| v69a.ibs * IBIS 4.1 Model
| 2Gb DDR-3 SDRAM - Die Revision "D"
| This Model is valid for Commercial Temperature Range (0C to 95C)
| Valid for DDR3-800/1066/1333/1600/1866/2133 operation
| Models *_1066 are applicable for speed grade 800/1066 Mbps
| Models *_1333 are applicable for speed grade 1333Mbps
| Models *_1600 are applicable for speed grade 1600Mbps
| Models *_2133 are applicable for speed grade 1866/2133 Mbps
| Part Number   VDD/VDDQ   Architecture   Package
| MT41J512M4HX   1.5V/1.5V   512Meg x 4   78-Ball 9x11.5 FBGA
| MT41J256M8HX   1.5V/1.5V   256Meg x 8   78-Ball 9x11.5 FBGA
| MT41J128M16HA   1.5V/1.5V   128Meg x 16   96-Ball 9x14.0 FBGA
| MT41J512M4V69A   1.5V/1.5V   512Meg x 4   Bare Die
| MT41J256M8V69A   1.5V/1.5V   256Meg x 8   Bare Die
| MT41J128M16V69A   1.5V/1.5V   128Meg x 16   Bare Die
[IBIS Ver]   4.2
[File name]   v69a.ibs
[Date]   05/11/2010
[File Rev]   2.1
[Source]   From silicon level SPICE model at Micron Technology, Inc.
   Micron Technology, Inc.
   8000 S. Federal Way
   P.O. Box 6, M/S: 01-711
   Boise, ID 83707-0006
   For support e-mail modelsupport@micron.com
[Notes]   Revision History:
   Rev 1.0: 05/01/2009
   - Initial pre-silicon model
   - Model data extracted from HSPICE model revision 1.0 (05/01/09)
   - Typ and slow corner V-t curves in the following DQ* models
   are shifted relative to strong corner v-t curve
   to contain all 3 corners within appropriate v-t window
   Models   Typ   Slow   v-t duration
   DQ*_1066   -250ps   -750ps   938ps
   DQ*_1333   -250ps   -750ps   750ps
   DQ*_1600   -290ps   -470ps   625ps
   DQ*_1866   -70ps   -140ps   468ps
   - Due to the shift in typ and slow corner, the v-t curves
   may overlap each other. This does not effect the accuracy
   of the ibis data.
   - For *_1600 models min (slow) corner uses typical process
   models
   - For *_1866 models typ(typ) and min (slow) corners uses
   fast process models
   - IQ SUMMARY Overall Quality of component and models Level 2b
   See Micron IBIS Model Quality Report for full IQ SUMMARY
   - This IBIS file uses the [Submodel] keyword to model the
   DDR-3 On-die Termination(ODT) characteristics.
   - The C_comp value in the DQ model is set to match the input
   state of the DQ I/O as measured from the HSPICE model.
   Due to the C_comp differences between the DQ model and the
   DQ_ODT* models, the output characteristics of the
   models will look different when simulated. To match most
   closely with the HSPICE model, simulate with the DQ_34
   or DQ_40 model for ALL Output simulations.  Use the ODT
   models ONLY for Input simulations.
   - All Submodels: when running through ibischk4.1, this file
   contains warnings about GND and Power Clamp data being
   non-monotonic. When Submodel I-V curves are added to
   non-odt Power and GND Clamp curves, the resultant
   curve is monotonic. This is not checked correctly with the
   IBIS parser.
   - Differential Receiver Thresholds in CLKIN* and DQS* models
   are commented out as it generates error when running through
   older ibischk parser.
   Rev 2.0: 01/25/2010
   - Model *_1066 and *_1333 are matched to measurement.
   - Model data extracted from HSPICE model revision 2.0 (01/25/2010)
   - Typ and slow corner V-t curves in the following DQ* models
   are shifted relative to strong corner v-t curve
   to contain all 3 corners within appropriate v-t window
   Models   Typ   Slow   v-t duration
   DQ*_1066   -200ps   -500ps   938ps
   DQ*_1333   -240ps   -600ps   750ps
   DQ*_1600   -240ps   -370ps   625ps
   DQ*_2133   -90ps   -190ps   469ps
   - Due to the shift in typ and slow corner, the v-t curves
   may overlap each other. This does not effect the accuracy
   of the ibis data.
   - For *_1600 models min (slow) corner uses typical process
   models
   - For *_2133 models typ(typ) and min (slow) corners uses
   fast process models
   -DQS* and CLKIN* models use differential [Receiver Thresholds]
   keyword which is supported in the latest IBIS 4.0 parser.
   This keywords may produce error when checked with older IBIS parser
   Please comment these keyword if your EDA simulation tool uses older
   IBISCHK parser
   - IQ SUMMARY Overall Quality of component and models Level 2b
   See Micron IBIS Model Quality Report for full IQ SUMMARY
   Rev 2.1: 05/11/2010
   - Added [Pin Mapping] sub-section for [Component]  section
   - Corrected vdiff in [Diff_pin] from 0.400V to 0.350V
[Disclaimer]  This software code and all associated documentation, comments
   or other information (collectively "Software") is provided
   "AS IS" without warranty of any kind. MICRON TECHNOLOGY, INC.
   ("MTI") EXPRESSLY DISCLAIMS ALL WARRANTIES EXPRESS OR IMPLIED,
   INCLUDING BUT NOT LIMITED TO, NONINFRINGEMENT OF THIRD PARTY
   RIGHTS, AND ANY IMPLIED WARRANTIES OF MERCHANTABILITY OR
   FITNESS FOR ANY PARTICULAR PURPOSE. MTI DOES NOT WARRANT THAT
   THE SOFTWARE WILL MEET YOUR REQUIREMENTS, OR THAT THE
   OPERATION OF THE SOFTWARE WILL BE UNINTERRUPTED OR ERROR-FREE.
   FURTHERMORE, MTI DOES NOT MAKE ANY REPRESENTATIONS REGARDING
   THE USE OR THE RESULTS OF THE USE OF THE SOFTWARE IN TERMS OF
   ITS CORRECTNESS, ACCURACY, RELIABILITY, OR OTHERWISE. THE
   ENTIRE RISK ARISING OUT OF USE OR PERFORMANCE OF THE SOFTWARE
   REMAINS WITH YOU. IN NO EVENT SHALL MTI, ITS AFFILIATED
   COMPANIES OR THEIR SUPPLIERS BE LIABLE FOR ANY DIRECT,
   INDIRECT, CONSEQUENTIAL, INCIDENTAL, OR SPECIAL DAMAGES
   (INCLUDING, WITHOUT LIMITATION, DAMAGES FOR LOSS OF PROFITS,
   BUSINESS INTERRUPTION, OR LOSS OF INFORMATION) ARISING OUT OF
   YOUR USE OF OR INABILITY TO USE THE SOFTWARE, EVEN IF MTI HAS
   BEEN ADVISED OF THE POSSIBILITY OF SUCH DAMAGES. Because some
   jurisdictions prohibit the exclusion or limitation of
   liability for consequential or incidental damages, the above
   limitation may not apply to you.
[Copyright]   Copyright 2008 Micron Technology, Inc. All rights reserved.
| COMPONENT: MT41J512M4HX (78-Ball FBGA, x4, 9mm X 11.5mm)
[Component]   MT41J512M4HX
[Package Model] V69A_X4_X8_FULL_PKG
[Manufacturer]  Micron Technology,Inc.
[Package]
|   typ   min   max
R_pkg   251.15m   182.00m   351.00m
L_pkg   1.57nH   1.09nH   2.34nH
C_pkg   0.37pF   0.26pF   0.50pF
[Pin]   signal_name model_name   R_pin   L_pin   C_pin
A1   VSS   GND
A2   VDD   POWER
A3   NC   NC
A7   NF   NF_INPUT   279.00m   1.35nH   0.42pF
A8   VSS   GND
A9   VDD   POWER
B1   VSS   GND
B2   VSSQ   GND
B3   DQ0   DQ   254.00m   1.10nH   0.38pF
B7   DM   DM   247.00m   2.19nH   0.37pF
B8   VSSQ   GND
B9   VDDQ   POWER
C1   VDDQ   POWER
C2   DQ2   DQ   330.00m   1.26nH   0.47pF
C3   DQS   DQS   263.00m   1.24nH   0.39pF
C7   DQ1   DQ   244.00m   1.33nH   0.37pF
C8   DQ3   DQ   340.00m   1.70nH   0.50pF
C9   VSSQ   GND
D1   VSSQ   GND
D2   NF   NF_INPUT   337.00m   1.93nH   0.49pF
D3   DQS#   DQS   244.00m   1.40nH   0.37pF
D7   VDD   POWER
D8   VSS   GND
D9   VSSQ   GND
E1   VREFDQ   POWER
E2   VDDQ   POWER
E3   NF   NF_INPUT   235.00m   1.79nH   0.36pF
E7   NF   NF_INPUT   209.00m   1.82nH   0.32pF
E8   NF   NF_INPUT   305.00m   1.76nH   0.45pF
E9   VDDQ   POWER
F1   NC   NC
F2   VSS   GND
F3   RAS#   INPUT   208.00m   1.39nH   0.32pF
F7   CK   CLKIN   234.00m   1.32nH   0.36pF
F8   VSS   GND
F9   NC   NC
G1   ODT   ODT_INPUT   335.00m   2.34nH   0.49pF
G2   VDD   POWER
G3   CAS#   INPUT   197.00m   1.33nH   0.29pF
G7   CK#   CLKIN   229.00m   1.36nH   0.32pF
G8   VDD   POWER
G9   CKE   INPUT   336.00m   2.21nH   0.48pF
H1   NC   NC
H2   CS#   INPUT   262.00m   1.81nH   0.36pF
H3   WE#   INPUT   188.00m   1.24nH   0.26pF
H7   A10   INPUT   195.00m   1.24nH   0.27pF
H8   ZQ   NC   268.00m   1.56nH   0.41pF
H9   NC   NC
J1   VSS   GND
J2   BA0   INPUT   262.00m   1.41nH   0.39pF
J3   BA2   INPUT   196.00m   1.12nH   0.30pF
J7   NC   NC
J8   VREFCA   POWER
J9   VSS   GND
K1   VDD   POWER
K2   A3   INPUT   255.00m   1.70nH   0.37pF
K3   A0   INPUT   189.00m   1.10nH   0.28pF
K7   A12   INPUT   182.00m   1.09nH   0.27pF
K8   BA1   INPUT   259.00m   1.75nH   0.37pF
K9   VDD   POWER
L1   VSS   GND
L2   A5   INPUT   255.00m   1.76nH   0.37pF
L3   A2   INPUT   183.00m   1.26nH   0.26pF
L7   A1   INPUT   184.00m   1.33nH   0.26pF
L8   A4   INPUT   250.00m   1.79nH   0.36pF
L9   VSS   GND
M1   VDD   POWER
M2   A7   INPUT   273.00m   1.82nH   0.40pF
M3   A9   INPUT   204.00m   1.40nH   0.31pF
M7   A11   INPUT   192.00m   1.35nH   0.28pF
M8   A6   INPUT   271.00m   1.93nH   0.40pF
M9   VDD   POWER
N1   VSS   GND
N2   RST#   INPUT   351.00m   1.98nH   0.50pF
N3   A13   INPUT   255.00m   1.67nH   0.37pF
N7   A14   INPUT   249.00m   1.49nH   0.37pF
N8   A8   INPUT   314.00m   2.19nH   0.44pF
N9   VSS   GND
|***********************PIN MAPPING*****************************************
[Pin Mapping] pulldown_ref pullup_ref gnd_clamp_ref power_clamp_ref ext_ref
A1   GNDBUS1   NC   |GNDBUS1 is VSS
A2   NC   PWRBUS1  |PWRBUS1 is VDD
A3   NC   NC
A7   NC   NC
A8   GNDBUS1   NC
A9   NC   PWRBUS1
B1   GNDBUS1   NC
B2   GNDBUS2   NC
B3   GNDBUS2   PWRBUS2   GNDBUS2   PWRBUS2
B7   GNDBUS2   PWRBUS2   GNDBUS2   PWRBUS2
B8   GNDBUS2   NC
B9   NC   PWRBUS2
C1   NC   PWRBUS2
C2   GNDBUS2   PWRBUS2   GNDBUS2   PWRBUS2 |GNDBUS2 is VSSQ
C3   GNDBUS2   PWRBUS2   GNDBUS2   PWRBUS2 |PWRBUS2 is VDDQ
C7   GNDBUS2   PWRBUS2   GNDBUS2   PWRBUS2
C8   GNDBUS2   PWRBUS2   GNDBUS2   PWRBUS2
C9   GNDBUS2   NC
D1   GNDBUS2   NC
D2   NC   NC
D3   GNDBUS2   PWRBUS2   GNDBUS2   PWRBUS2
D7   NC   PWRBUS1
D8   GNDBUS1   NC
D9   GNDBUS2   NC
E1   NC   REFDQ   |VREFDQ
E2   NC   PWRBUS2
E3   NC   NC
E7   NC   NC
E8   NC   NC
E9   NC   PWRBUS2
F1   NC   NC
F2   GNDBUS1   NC
F3   GNDBUS1   PWRBUS1   GNDBUS1   PWRBUS1
F7   GNDBUS1   PWRBUS1   GNDBUS1   PWRBUS1
F8   GNDBUS1   NC
F9   NC   NC
G1   GNDBUS1   PWRBUS1   GNDBUS1   PWRBUS1
G2   NC   PWRBUS1
G3   GNDBUS1   PWRBUS1   GNDBUS1   PWRBUS1
G7   GNDBUS1   PWRBUS1   GNDBUS1   PWRBUS1
G8   NC   PWRBUS1
G9   GNDBUS1   PWRBUS1   GNDBUS1   PWRBUS1
H1   NC   NC
H2   GNDBUS1   PWRBUS1   GNDBUS1   PWRBUS1
H3   GNDBUS1   PWRBUS1   GNDBUS1   PWRBUS1
H7   GNDBUS1   PWRBUS1   GNDBUS1   PWRBUS1
H8   NC   NC
H9   NC   NC
J1   GNDBUS1   NC
J2   GNDBUS1   PWRBUS1   GNDBUS1   PWRBUS1
J3   GNDBUS1   PWRBUS1   GNDBUS1   PWRBUS1
J7   NC   NC
J8   NC   REFCA   |VREFCA
J9   GNDBUS1   NC
K1   NC   PWRBUS1
K2   GNDBUS1   PWRBUS1   GNDBUS1   PWRBUS1
K3   GNDBUS1   PWRBUS1   GNDBUS1   PWRBUS1
K7   GNDBUS1   PWRBUS1   GNDBUS1   PWRBUS1
K8   GNDBUS1   PWRBUS1   GNDBUS1   PWRBUS1
K9   NC   PWRBUS1
L1   GNDBUS1   NC
L2   GNDBUS1   PWRBUS1   GNDBUS1   PWRBUS1
L3   GNDBUS1   PWRBUS1   GNDBUS1   PWRBUS1
L7   GNDBUS1   PWRBUS1   GNDBUS1   PWRBUS1
L8   GNDBUS1   PWRBUS1   GNDBUS1   PWRBUS1
L9   GNDBUS1   NC
M1   NC   PWRBUS1
M2   GNDBUS1   PWRBUS1   GNDBUS1   PWRBUS1
M3   GNDBUS1   PWRBUS1   GNDBUS1   PWRBUS1
M7   GNDBUS1   PWRBUS1   GNDBUS1   PWRBUS1
M8   GNDBUS1   PWRBUS1   GNDBUS1   PWRBUS1
M9   NC   PWRBUS1
N1   GNDBUS1   NC
N2   GNDBUS1   PWRBUS1   GNDBUS1   PWRBUS1
N3   GNDBUS1   PWRBUS1   GNDBUS1   PWRBUS1
N7   GNDBUS1   PWRBUS1   GNDBUS1   PWRBUS1
N8   GNDBUS1   PWRBUS1   GNDBUS1   PWRBUS1
N9   GNDBUS1   NC
|**********************DIFF PIN*********************************************
[Diff_pin]   inv_pin   vdiff   tdelay_typ   tdelay_min   tdelay_max
   C3   D3   0.350V   0ns   NA   NA
   F7   G7   0.350V   0ns   NA   NA
| COMPONENT: MT41J256M8HX (78-Ball FBGA, x8, 9mm X 11.5mm)
[Component]  MT41J256M8HX
[Package Model] V69A_X4_X8_FULL_PKG
[Manufacturer]  Micron Technology,Inc.
[Package]
|   typ   min   max
R_pkg   251.15m   182.00m   351.00m
L_pkg   1.57nH   1.09nH   2.34nH
C_pkg   0.37pF   0.26pF   0.50pF
[Pin]   signal_name model_name   R_pin   L_pin   C_pin
A1   VSS   GND
A2   VDD   POWER
A3   NC   NC
A7   NF_TDQS#   NF_TDQS#   279.00m   1.35nH   0.42pF
A8   VSS   GND
A9   VDD   POWER
B1   VSS   GND
B2   VSSQ   GND
B3   DQ0   DQ   254.00m   1.10nH   0.38pF
B7   DM_TDQS   DM_TDQS   247.00m   2.19nH   0.37pF
B8   VSSQ   GND
B9   VDDQ   POWER
C1   VDDQ   POWER
C2   DQ2   DQ   330.00m   1.26nH   0.47pF
C3   DQS   DQS   263.00m   1.24nH   0.39pF
C7   DQ1   DQ   244.00m   1.33nH   0.37pF
C8   DQ3   DQ   340.00m   1.70nH   0.50pF
C9   VSSQ   GND
D1   VSSQ   GND
D2   DQ6   DQ   337.00m   1.93nH   0.49pF
D3   DQS#   DQS   244.00m   1.40nH   0.37pF
D7   VDD   POWER
D8   VSS   GND
D9   VSSQ   GND
E1   VREFDQ   POWER
E2   VDDQ   POWER
E3   DQ4   DQ   235.00m   1.79nH   0.36pF
E7   DQ7   DQ   209.00m   1.82nH   0.32pF
E8   DQ5   DQ   305.00m   1.76nH   0.45pF
E9   VDDQ   POWER
F1   NC   NC
F2   VSS   GND
F3   RAS#   INPUT   208.00m   1.39nH   0.32pF
F7   CK   CLKIN   234.00m   1.32nH   0.36pF
F8   VSS   GND
F9   NC   NC
G1   ODT   ODT_INPUT   335.00m   2.34nH   0.49pF
G2   VDD   POWER
G3   CAS#   INPUT   197.00m   1.33nH   0.29pF
G7   CK#   CLKIN   229.00m   1.36nH   0.32pF
G8   VDD   POWER
G9   CKE   INPUT   336.00m   2.21nH   0.48pF
H1   NC   NC
H2   CS#   INPUT   262.00m   1.81nH   0.36pF
H3   WE#   INPUT   188.00m   1.24nH   0.26pF
H7   A10   INPUT   195.00m   1.24nH   0.27pF
H8   ZQ   NC   268.00m   1.56nH   0.41pF
H9   NC   NC
J1   VSS   GND
J2   BA0   INPUT   262.00m   1.41nH   0.39pF
J3   BA2   INPUT   196.00m   1.12nH   0.30pF
J7   NC   NC
J8   VREFCA   POWER
J9   VSS   GND
K1   VDD   POWER
K2   A3   INPUT   255.00m   1.70nH   0.37pF
K3   A0   INPUT   189.00m   1.10nH   0.28pF
K7   A12   INPUT   182.00m   1.09nH   0.27pF
K8   BA1   INPUT   259.00m   1.75nH   0.37pF
K9   VDD   POWER
L1   VSS   GND
L2   A5   INPUT   255.00m   1.76nH   0.37pF
L3   A2   INPUT   183.00m   1.26nH   0.26pF
L7   A1   INPUT   184.00m   1.33nH   0.26pF
L8   A4   INPUT   250.00m   1.79nH   0.36pF
L9   VSS   GND
M1   VDD   POWER
M2   A7   INPUT   273.00m   1.82nH   0.40pF
M3   A9   INPUT   204.00m   1.40nH   0.31pF
M7   A11   INPUT   192.00m   1.35nH   0.28pF
M8   A6   INPUT   271.00m   1.93nH   0.40pF
M9   VDD   POWER
N1   VSS   GND
N2   RST#   INPUT   351.00m   1.98nH   0.50pF
N3   A13   INPUT   255.00m   1.67nH   0.37pF
N7   A14   INPUT   249.00m   1.49nH   0.37pF
N8   A8   INPUT   314.00m   2.19nH   0.44pF
N9   VSS   GND
|***********************PIN MAPPING*****************************************
[Pin Mapping] pulldown_ref pullup_ref gnd_clamp_ref power_clamp_ref ext_ref
A1   GNDBUS1   NC   |GNDBUS1 is VSS
A2   NC   PWRBUS1   |PWRBUS1 is VDD
A3   NC   NC
A7   GNDBUS2   PWRBUS2   GNDBUS2   PWRBUS2   |PWRBUS2 is VDDQ
A8   GNDBUS1   NC
A9   NC   PWRBUS1
B1   GNDBUS1   NC
B2   GNDBUS2   NC
B3   GNDBUS2   PWRBUS2   GNDBUS2   PWRBUS2   |GNDBUS2 is VSSQ
B7   GNDBUS2   PWRBUS2   GNDBUS2   PWRBUS2
B8   GNDBUS2   NC
B9   NC   PWRBUS2
C1   NC   PWRBUS2
C2   GNDBUS2   PWRBUS2   GNDBUS2   PWRBUS2
C3   GNDBUS2   PWRBUS2   GNDBUS2   PWRBUS2
C7   GNDBUS2   PWRBUS2   GNDBUS2   PWRBUS2
C8   GNDBUS2   PWRBUS2   GNDBUS2   PWRBUS2
C9   GNDBUS2   NC
D1   GNDBUS2   NC
D2   GNDBUS2   PWRBUS2   GNDBUS2   PWRBUS2
D3   GNDBUS2   PWRBUS2   GNDBUS2   PWRBUS2
D7   NC   PWRBUS1
D8   GNDBUS1   NC
D9   GNDBUS2   NC
E1   NC   REFDQ   |VREFDQ
E2   NC   PWRBUS2
E3   GNDBUS2   PWRBUS2   GNDBUS2   PWRBUS2
E7   GNDBUS2   PWRBUS2   GNDBUS2   PWRBUS2
E8   GNDBUS2   PWRBUS2   GNDBUS2   PWRBUS2
E9   NC   PWRBUS2
F1   NC   NC
F2   GNDBUS1   NC
F3   GNDBUS1   PWRBUS1   GNDBUS1   PWRBUS1
F7   GNDBUS1   PWRBUS1   GNDBUS1   PWRBUS1
F8   GNDBUS1   NC
F9   NC   NC
G1   GNDBUS1   PWRBUS1   GNDBUS1   PWRBUS1
G2   NC   PWRBUS1
G3   GNDBUS1   PWRBUS1   GNDBUS1   PWRBUS1
G7   GNDBUS1   PWRBUS1   GNDBUS1   PWRBUS1
G8   NC   PWRBUS1
G9   GNDBUS1   PWRBUS1   GNDBUS1   PWRBUS1
H1   NC   NC
H2   GNDBUS1   PWRBUS1   GNDBUS1   PWRBUS1
H3   GNDBUS1   PWRBUS1   GNDBUS1   PWRBUS1
H7   GNDBUS1   PWRBUS1   GNDBUS1   PWRBUS1
H8   NC   NC
H9   NC   NC
J1   GNDBUS1   NC
J2   GNDBUS1   PWRBUS1   GNDBUS1   PWRBUS1
J3   GNDBUS1   PWRBUS1   GNDBUS1   PWRBUS1
J7   NC   NC
J8   NC   REFCA   |VREFCA
J9   GNDBUS1   NC
K1   NC   PWRBUS1
K2   GNDBUS1   PWRBUS1   GNDBUS1   PWRBUS1
K3   GNDBUS1   PWRBUS1   GNDBUS1   PWRBUS1
K7   GNDBUS1   PWRBUS1   GNDBUS1   PWRBUS1
K8   GNDBUS1   PWRBUS1   GNDBUS1   PWRBUS1
K9   NC   PWRBUS1
L1   GNDBUS1   NC
L2   GNDBUS1   PWRBUS1   GNDBUS1   PWRBUS1
L3   GNDBUS1   PWRBUS1   GNDBUS1   PWRBUS1
L7   GNDBUS1   PWRBUS1   GNDBUS1   PWRBUS1
L8   GNDBUS1   PWRBUS1   GNDBUS1   PWRBUS1
L9   GNDBUS1   NC
M1   NC   PWRBUS1
M2   GNDBUS1   PWRBUS1   GNDBUS1   PWRBUS1
M3   GNDBUS1   PWRBUS1   GNDBUS1   PWRBUS1
M7   GNDBUS1   PWRBUS1   GNDBUS1   PWRBUS1
M8   GNDBUS1   PWRBUS1   GNDBUS1   PWRBUS1
M9   NC   PWRBUS1
N1   GNDBUS1   NC
N2   GNDBUS1   PWRBUS1   GNDBUS1   PWRBUS1
N3   GNDBUS1   PWRBUS1   GNDBUS1   PWRBUS1
N7   GNDBUS1   PWRBUS1   GNDBUS1   PWRBUS1
N8   GNDBUS1   PWRBUS1   GNDBUS1   PWRBUS1
N9   GNDBUS1   NC
|**********************DIFF PIN*********************************************
[Diff_pin]   inv_pin   vdiff   tdelay_typ   tdelay_min   tdelay_max
   C3   D3   0.350V   0ns   NA   NA
   F7   G7   0.350V   0ns   NA   NA
| COMPONENT: MT41J128M16HA (96-Ball FBGA, x16, 9mm X 14mm)
[Component]   MT41J128M16HA
[Package Model] V69A_X16_FULL_PKG
[Manufacturer]  Micron Technology,Inc.
[Package]
|   typ   min   max
R_pkg   265.65m   194.00m   421.00m
L_pkg   1.43nH   0.93nH   2.58nH
C_pkg   0.40pF   0.30pF   0.60pF
[Pin]   signal_name model_name   R_pin   L_pin   C_pin
A1   VDDQ   POWER
A2   DQ13   DQ   340.00m   1.53nH   0.52pF
A3   DQ15   DQ   260.00m   1.29nH   0.40pF
A7   DQ12   DQ   235.00m   1.19nH   0.38pF
A8   VDDQ   POWER
A9   VSS   GND
B1   VSSQ   GND
B2   VDD   POWER
B3   VSS   GND
B7   UDQS#   DQS   245.00m   1.18nH   0.38pF
B8   DQ14   DQ   317.00m   1.41nH   0.49pF
B9   VSSQ   GND
C1   VDDQ   POWER
C2   DQ11   DQ   301.00m   1.30nH   0.46pF
C3   DQ9   DQ   223.00m   1.07nH   0.36pF
C7   UDQS   DQS   225.00m   1.09nH   0.36pF
C8   DQ10   DQ   313.00m   1.31nH   0.47pF
C9   VDDQ   POWER
D1   VSSQ   GND
D2   VDDQ   POWER
D3   UDM   DM   218.00m   1.24nH   0.33pF
D7   DQ8   DQ   209.00m   0.96nH   0.34pF
D8   VSSQ   GND
D9   VDD   POWER
E1   VSS   GND
E2   VSSQ   GND
E3   DQ0   DQ   204.00m   1.02nH   0.33pF
E7   LDM   DM   195.00m   1.10nH   0.31pF
E8   VSSQ   GND
E9   VDDQ   POWER
F1   VDDQ   POWER
F2   DQ2   DQ   285.00m   1.30nH   0.43pF
F3   LDQS   DQS   234.00m   1.12nH   0.37pF
F7   DQ1   DQ   198.00m   0.96nH   0.32pF
F8   DQ3   DQ   284.00m   1.23nH   0.44pF
F9   VSSQ   GND
G1   VSSQ   GND
G2   DQ6   DQ   284.00m   1.23nH   0.43pF
G3   LDQS#   DQS   234.00m   1.11nH   0.37pF
G7   VDD   POWER
G8   VSS   GND
G9   VSSQ   GND
H1   VREFDQ   POWER
H2   VDDQ   POWER
H3   DQ4   DQ   194.00m   0.93nH   0.31pF
H7   DQ7   DQ   201.00m   1.00nH   0.33pF
H8   DQ5   DQ   271.00m   1.15nH   0.42pF
H9   VDDQ   POWER
J1   NC   NC
J2   VSS   GND
J3   RAS#   INPUT   198.00m   1.14nH   0.32pF
J7   CK   CLKIN   218.00m   1.15nH   0.34pF
J8   VSS   GND
J9   NC   NC
K1   ODT   ODT_INPUT   353.00m   1.14nH   0.52pF
K2   VDD   POWER
K3   CAS#   INPUT   205.00m   1.06nH   0.30pF
K7   CK#   CLKIN   215.00m   1.24nH   0.33pF
K8   VDD   POWER
K9   CKE   INPUT   369.00m   2.33nH   0.53pF
L1   NC   NC
L2   CS#   INPUT   274.00m   1.80nH   0.39pF
L3   WE#   INPUT   213.00m   1.33nH   0.31pF
L7   A10   INPUT   207.00m   1.24nH   0.31pF
L8   ZQ   NC   298.00m   1.62nH   0.46pF
L9   NC   NC
M1   VSS   GND
M2   BA0   INPUT   297.00m   1.48nH   0.43pF
M3   BA2   INPUT   200.00m   1.09nH   0.30pF
M7   NC   NC
M8   VREFCA   POWER
M9   VSS   GND
N1   VDD   POWER
N2   A3   INPUT   302.00m   1.86nH   0.45pF
N3   A0   INPUT   214.00m   1.14nH   0.33pF
N7   A12   INPUT   233.00m   1.33nH   0.36pF
N8   BA1   INPUT   326.00m   1.98nH   0.48pF
N9   VDD   POWER
P1   VSS   GND
P2   A5   INPUT   300.00m   1.94nH   0.44pF
P3   A2   INPUT   231.00m   1.53nH   0.34pF
P7   A1   INPUT   245.00m   1.65nH   0.37pF
P8   A4   INPUT   323.00m   2.07nH   0.48pF
P9   VSS   GND
R1   VDD   POWER
R2   A7   INPUT   338.00m   2.21nH   0.50pF
R3   A9   INPUT   271.00m   1.81nH   0.40pF
R7   A11   INPUT   268.00m   1.74nH   0.39pF
R8   A6   INPUT   346.00m   2.32nH   0.50pF
R9   VDD   POWER
T1   VSS   GND
T2   RST#   INPUT   421.00m   1.65nH   0.60pF
T3   A13   INPUT   322.00m   2.11nH   0.47pF
T7   NC   NC
T8   A8   INPUT   392.00m   2.58nH   0.57pF
T9   VSS   GND
|***********************PIN MAPPING*****************************************
[Pin Mapping] pulldown_ref pullup_ref gnd_clamp_ref power_clamp_ref ext_ref
A1   NC   PWRBUS2   |PWRBUS1 is VDD
A2   GNDBUS2   PWRBUS2   GNDBUS2   PWRBUS2 |PWRBUS2 is VDDQ
A3   GNDBUS2   PWRBUS2   GNDBUS2   PWRBUS2 |GNDBUS2 is VSSQ
A7   GNDBUS2   PWRBUS2   GNDBUS2   PWRBUS2
A8   NC   PWRBUS2
A9   GNDBUS1   NC
B1   GNDBUS2   NC
B2   NC   PWRBUS1   |GNDBUS1 is VSS
B3   GNDBUS1   NC
B7   GNDBUS2   PWRBUS2   GNDBUS2   PWRBUS2
B8   GNDBUS2   PWRBUS2   GNDBUS2   PWRBUS2
B9   GNDBUS2   NC
C1   NC   PWRBUS2
C2   GNDBUS2   PWRBUS2   GNDBUS2   PWRBUS2
C3   GNDBUS2   PWRBUS2   GNDBUS2   PWRBUS2
C7   GNDBUS2   PWRBUS2   GNDBUS2   PWRBUS2
C8   GNDBUS2   PWRBUS2   GNDBUS2   PWRBUS2
C9   NC   PWRBUS2
D1   GNDBUS2   NC
D2   NC   PWRBUS2
D3   GNDBUS2   PWRBUS2   GNDBUS2   PWRBUS2
D7   GNDBUS2   PWRBUS2   GNDBUS2   PWRBUS2
D8   GNDBUS2   NC
D9   NC   PWRBUS1
E1   GNDBUS1   NC
E2   GNDBUS2   NC
E3   GNDBUS2   PWRBUS2   GNDBUS2   PWRBUS2
E7   GNDBUS2   PWRBUS2   GNDBUS2   PWRBUS2
E8   GNDBUS2   NC
E9   NC   PWRBUS2
F1   NC   PWRBUS2
F2   GNDBUS2   PWRBUS2   GNDBUS2   PWRBUS2
F3   GNDBUS2   PWRBUS2   GNDBUS2   PWRBUS2
F7   GNDBUS2   PWRBUS2   GNDBUS2   PWRBUS2
F8   GNDBUS2   PWRBUS2   GNDBUS2   PWRBUS2
F9   GNDBUS2   NC
G1   GNDBUS2   NC
G2   GNDBUS2   PWRBUS2   GNDBUS2   PWRBUS2
G3   GNDBUS2   PWRBUS2   GNDBUS2   PWRBUS2
G7   NC   PWRBUS1
G8   GNDBUS1   NC
G9   GNDBUS2   NC
H1   NC   REFDQ   |VREFDQ
H2   NC   PWRBUS2
H3   GNDBUS2   PWRBUS2   GNDBUS2   PWRBUS2
H7   GNDBUS2   PWRBUS2   GNDBUS2   PWRBUS2
H8   GNDBUS2   PWRBUS2   GNDBUS2   PWRBUS2
H9   NC   PWRBUS2
J1   NC   NC
J2   GNDBUS1   NC
J3   GNDBUS1   PWRBUS1   GNDBUS1   PWRBUS1
J7   GNDBUS1   PWRBUS1   GNDBUS1   PWRBUS1
J8   GNDBUS1   NC
J9   NC   NC
K1   GNDBUS1   PWRBUS1   GNDBUS1   PWRBUS1
K2   NC   PWRBUS1
K3   GNDBUS1   PWRBUS1   GNDBUS1   PWRBUS1
K7   GNDBUS1   PWRBUS1   GNDBUS1   PWRBUS1
K8   NC   PWRBUS1
K9   GNDBUS1   PWRBUS1   GNDBUS1   PWRBUS1
L1   NC   NC
L2   GNDBUS1   PWRBUS1   GNDBUS1   PWRBUS1
L3   GNDBUS1   PWRBUS1   GNDBUS1   PWRBUS1
L7   GNDBUS1   PWRBUS1   GNDBUS1   PWRBUS1
L8   NC   NC
L9   NC   NC
M1   GNDBUS1   NC
M2   GNDBUS1   PWRBUS1   GNDBUS1   PWRBUS1
M3   GNDBUS1   PWRBUS1   GNDBUS1   PWRBUS1
M7   NC   NC
M8   NC   REFCA   |VREFCA
M9   GNDBUS1   NC
N1   NC   PWRBUS1
N2   GNDBUS1   PWRBUS1   GNDBUS1   PWRBUS1
N3   GNDBUS1   PWRBUS1   GNDBUS1   PWRBUS1
N7   GNDBUS1   PWRBUS1   GNDBUS1   PWRBUS1
N8   GNDBUS1   PWRBUS1   GNDBUS1   PWRBUS1
N9   NC   PWRBUS1
P1   GNDBUS1   NC
P2   GNDBUS1   PWRBUS1   GNDBUS1   PWRBUS1
P3   GNDBUS1   PWRBUS1   GNDBUS1   PWRBUS1
P7   GNDBUS1   PWRBUS1   GNDBUS1   PWRBUS1
P8   GNDBUS1   PWRBUS1   GNDBUS1   PWRBUS1
P9   GNDBUS1   NC
R1   NC   PWRBUS1
R2   GNDBUS1   PWRBUS1   GNDBUS1   PWRBUS1
R3   GNDBUS1   PWRBUS1   GNDBUS1   PWRBUS1
R7   GNDBUS1   PWRBUS1   GNDBUS1   PWRBUS1
R8   GNDBUS1   PWRBUS1   GNDBUS1   PWRBUS1
R9   NC   PWRBUS1
T1   GNDBUS1   NC
T2   GNDBUS1   PWRBUS1   GNDBUS1   PWRBUS1
T3   GNDBUS1   PWRBUS1   GNDBUS1   PWRBUS1
T7   NC   NC
T8   GNDBUS1   PWRBUS1   GNDBUS1   PWRBUS1
T9   GNDBUS1   NC
|**********************DIFF PIN*********************************************
[Diff_pin]   inv_pin   vdiff   tdelay_typ   tdelay_min   tdelay_max
   F3   G3   0.350V   0ns   NA   NA
   C7   B7   0.350V   0ns   NA   NA
   J7   K7   0.350V   0ns   NA   NA
| COMPONENT: MT41J512M4V69A (Bare Die, x4)
[Component]   MT41J512M4V69A
[Manufacturer]  Micron Technology, Inc.
[Package]
|variable   typ   min   max
R_pkg   0.001m   0.001m   0.001m
L_pkg   0.001nH   0.001nH   0.001nH
C_pkg   0.001pF   0.001pF   0.001pF
[Pin]  signal_name   model_name   R_pin   L_pin   C_pin
1   VDD   POWER
2   DNU   NC
3   DNU   NC
4   DNU   NC
5   VSS   GND
6   VDD   POWER
7   DNU   NC
8   VSS   GND
9   VDD   POWER
10   RESET#   INPUT
11   A14   INPUT
12   A13   INPUT
13   A11   INPUT
14   A9   INPUT
15   A7   INPUT
16   A8   INPUT
17   A2   INPUT
18   A6   INPUT
19   A5   INPUT
20   A1   INPUT
21   A3   INPUT
22   A4   INPUT
23   A0   INPUT
24   VSS   GND
25   VDD   POWER
26   BA1   INPUT
27   A12   INPUT
28   BA0   INPUT
29   BA2   INPUT
30   VDD   POWER
31   VSS   GND
32   DNU   NC
33   DNU   NC
34   VREFCA   POWER
35   DNU   NC
36   VDDQ   POWER
37   ZQ   INPUT
38   VSSQ   GND
39   A10   INPUT
40   VSS   GND
41   VDD   POWER
42   DNU   NC
43   DNU   NC
44   DNU   NC
45   WE   INPUT
46   CS   INPUT
47   ODT_INPUT   INPUT
48   DNU   NC
49   CKE   INPUT
50   DNU   NC
51   CK#   CLKIN
52   CK   CLKIN
53   VDD   POWER
54   VSS   GND
55   CAS   INPUT
56   VDDDLL   POWER
57   VSSDL   GND
58   RAS   INPUT
59   DNU   NC
60   VREFDQ   POWER
61   VSSQ   GND
62   DNU   NC
63   VDDQ   POWER
64   DNU   NC
65   VSSQ   GND
66   VSSQ   GND
67   DNU   NC
68   VDDQ   POWER
69   DNU   NC
70   VSS   GND
71   VSSQ   GND
72   VDD   POWER
73   VSS   GND
74   VSSQ   GND
75   DQS#   DQS
76   VDDQ   POWER
77   DQS   DQS
78   VSSQ   GND
79   VSSQ   GND
80   DQ1   DQ
81   VDDQ   POWER
82   DQ3   DQ
83   VSSQ   GND
84   VSSQ   GND
85   DQ2   DQ
86   VDDQ   POWER
87   DQ0   DQ
88   VSSQ   GND
89   DM   DM
90   VDD   POWER
91   VSS   GND
92   DNU   NC
93   VDDQ   POWER
94   DNU   NC
95   VSSQ   GND
96   DNU   NC
97   VDDQ   POWER
98   VDDQ   POWER
99   DNU   NC
100   VSSQ   GND
101   DNU   NC
102   VDDQ   POWER
103   VDDQ   POWER
104   DNU   NC
105   VSSQ   GND
106   DNU   NC
107   VDDQ   POWER
108   VDD   POWER
109   VSS   GND
110   VDDQ   POWER
111   DNU   NC
112   VSSQ   GND
113   DNU   NC
114   VDDQ   POWER
115   VDDQ   POWER
116   DNU   NC
117   VSSQ   GND
118   DNU   NC
119   VDDQ   POWER
120   DNU   NC
|**********************DIFF PIN*********************************************
[Diff_pin]   inv_pin   vdiff   tdelay_typ   tdelay_min   tdelay_max
   52   51   0.350V   0ns   NA   NA
   77   75   0.350V   0ns   NA   NA
| COMPONENT: MT41J256M8V69A (Bare Die, x8)
[Component]   MT41J256M8V69A
[Manufacturer]  Micron Technology, Inc.
[Package]
|variable   typ   min   max
R_pkg   0.001m   0.001m   0.001m
L_pkg   0.001nH   0.001nH   0.001nH
C_pkg   0.001pF   0.001pF   0.001pF
[Pin]  signal_name   model_name   R_pin   L_pin   C_pin
1   VDD   POWER
2   DNU   NC
3   DNU   NC
4   DNU   NC
5   VSS   GND
6   VDD   POWER
7   DNU   NC
8   VSS   GND
9   VDD   POWER
10   RESET#   INPUT
11   A14   INPUT
12   A13   INPUT
13   A11   INPUT
14   A9   INPUT
15   A7   INPUT
16   A8   INPUT
17   A2   INPUT
18   A6   INPUT
19   A5   INPUT
20   A1   INPUT
21   A3   INPUT
22   A4   INPUT
23   A0   INPUT
24   VSS   GND
25   VDD   POWER
26   BA1   INPUT
27   A12   INPUT
28   BA0   INPUT
29   BA2   INPUT
30   VDD   POWER
31   VSS   GND
32   DNU   NC
33   DNU   NC
34   VREFCA   POWER
35   DNU   NC
36   VDDQ   POWER
37   ZQ   INPUT
38   VSSQ   GND
39   A10   INPUT
40   VSS   GND
41   VDD   POWER
42   DNU   NC
43   DNU   NC
44   DNU   NC
45   WE   INPUT
46   CS   INPUT
47   ODT   ODT_INPUT
48   DNU   NC
49   CKE   INPUT
50   DNU   NC
51   CK#   CLKIN
52   CK   CLKIN
53   VDD   POWER
54   VSS   GND
55   CAS   INPUT
56   VDDDLL   POWER
57   VSSDL   GND
58   RAS   INPUT
59   DNU   NC
60   VREFDQ   POWER
61   VSSQ   GND
62   DQ4   DQ
63   VDDQ   POWER
64   DQ6   DQ
65   VSSQ   GND
66   VSSQ   GND
67   DQ7   DQ
68   VDDQ   POWER
69   DQ5   DQ
70   VSS   GND
71   VSSQ   GND
72   VDD   POWER
73   VSS   GND
74   VSSQ   GND
75   DQS#   DQS
76   VDDQ   POWER
77   DQS   DQS
78   VSSQ   GND
79   VSSQ   GND
80   DQ1   DQ
81   VDDQ   POWER
82   DQ3   DQ
83   VSSQ   GND
84   VSSQ   GND
85   DQ2   DQ
86   VDDQ   POWER
87   DQ0   DQ
88   VSSQ   GND
89   DM_TDQS   DM_TDQS
90   VDD   POWER
91   VSS   GND
92   NF_TDQS#   NF_TDQS#
93   VDDQ   POWER
94   DNU   NC
95   VSSQ   GND
96   DNU   NC
97   VDDQ   POWER
98   VDDQ   POWER
99   DNU   NC
100   VSSQ   GND
101   DNU   NC
102   VDDQ   POWER
103   VDDQ   POWER
104   DNU   NC
105   VSSQ   GND
106   DNU   NC
107   VDDQ   POWER
108   VDD   POWER
109   VSS   GND
110   VDDQ   POWER
111   DNU   NC
112   VSSQ   GND
113   DNU   NC
114   VDDQ   POWER
115   VDDQ   POWER
116   DNU   NC
117   VSSQ   GND
118   DNU   NC
119   VDDQ   POWER
120   DNU   NC
|**********************DIFF PIN*********************************************
[Diff_pin]   inv_pin   vdiff   tdelay_typ   tdelay_min   tdelay_max
   52   51   0.350V   0ns   NA   NA
   77   75   0.350V   0ns   NA   NA
| COMPONENT: MT41J128M16V69A (Bare Die, x16)
[Component]   MT41J128M16V69A
[Manufacturer]  Micron Technology, Inc.
[Package]
|variable   typ   min   max
R_pkg   0.001m   0.001m   0.001m
L_pkg   0.001nH   0.001nH   0.001nH
C_pkg   0.001pF   0.001pF   0.001pF
[Pin]  signal_name   model_name   R_pin   L_pin   C_pin
1   VDD   POWER
2   DNU   NC
3   DNU   NC
4   DNU   NC
5   VSS   GND
6   VDD   POWER
7   DNU   NC
8   VSS   GND
9   VDD   POWER
10   RESET#   INPUT
11   DNU   NC
12   A13   INPUT
13   A11   INPUT
14   A9   INPUT
15   A7   INPUT
16   A8   INPUT
17   A2   INPUT
18   A6   INPUT
19   A5   INPUT
20   A1   INPUT
21   A3   INPUT
22   A4   INPUT
23   A0   INPUT
24   VSS   GND
25   VDD   POWER
26   BA1   INPUT
27   A12   INPUT
28   BA0   INPUT
29   BA2   INPUT
30   VDD   POWER
31   VSS   GND
32   DNU   NC
33   DNU   NC
34   VREFCA   POWER
35   DNU   NC
36   VDDQ   POWER
37   ZQ   INPUT
38   VSSQ   GND
39   A10   INPUT
40   VSS   GND
41   VDD   POWER
42   DNU   NC
43   DNU   NC
44   DNU   NC
45   WE   INPUT
46   CS   INPUT
47   ODT   ODT_INPUT
48   DNU   NC
49   CKE   INPUT
50   DNU   NC
51   CK#   CLKIN
52   CK   CLKIN
53   VDD   POWER
54   VSS   GND
55   CAS   INPUT
56   VDDDLL   POWER
57   VSSDL   GND
58   RAS   INPUT
59   DNU   NC
60   VREFDQ   POWER
61   VSSQ   GND
62   DQ4   DQ
63   VDDQ   POWER
64   DQ6   DQ
65   VSSQ   GND
66   VSSQ   GND
67   DQ7   DQ
68   VDDQ   POWER
69   DQ5   DQ
70   VSS   GND
71   VSSQ   GND
72   VDD   POWER
73   VSS   GND
74   VSSQ   GND
75   LDQS#   DQS
76   VDDQ   POWER
77   LDQS   DQS
78   VSSQ   GND
79   VSSQ   GND
80   DQ1   DQ
81   VDDQ   POWER
82   DQ3   DQ
83   VSSQ   GND
84   VSSQ   GND
85   DQ2   DQ
86   VDDQ   POWER
87   DQ0   DQ
88   VSSQ   GND
89   LDM   DM
90   VDD   POWER
91   VSS   GND
92   UDM   DM
93   VDDQ   POWER
94   DQ8   DQ
95   VSSQ   GND
96   DQ10   DQ
97   VDDQ   POWER
98   VDDQ   POWER
99   DQ11   DQ
100   VSSQ   GND
101   DQ9   DQ
102   VDDQ   POWER
103   VDDQ   POWER
104   UDQS   DQS
105   VSSQ   GND
106   UDQS#   DQS
107   VDDQ   POWER
108   VDD   POWER
109   VSS   GND
110   VDDQ   POWER
111   DQ13   DQ
112   VSSQ   GND
113   DQ15   DQ
114   VDDQ   POWER
115   VDDQ   POWER
116   DQ14   DQ
117   VSSQ   GND
118   DQ12   DQ
119   VDDQ   POWER
120   DNU   NC
|**********************DIFF PIN*********************************************
[Diff_pin]   inv_pin   vdiff   tdelay_typ   tdelay_min   tdelay_max
   52   51   0.350V   0ns   NA   NA
   77   75   0.350V   0ns   NA   NA
   104   106   0.350V   0ns   NA   NA
|   Model Selector
[Model Selector] DQ
DQ_34_1066   34 Ohm Data I/O with no ODT (800/1066Mbps)
DQ_34_ODT20_1066   34 Ohm Data I/O with 20 Ohm ODT Submodel (800/1066Mbps)
DQ_34_ODT30_1066   34 Ohm Data I/O with 30 Ohm ODT Submodel (800/1066Mbps)
DQ_34_ODT40_1066   34 Ohm Data I/O with 40 Ohm ODT Submodel (800/1066Mbps)
DQ_34_ODT60_1066   34 Ohm Data I/O with 60 Ohm ODT Submodel (800/1066Mbps)
DQ_34_ODT120_1066  34 Ohm Data I/O with 120 Ohm ODT Submodel (800/1066Mbps)
DQ_40_1066   40 Ohm Data I/O with no ODT (800/1066Mbps)
DQ_40_ODT20_1066   40 Ohm Data I/O with 20 Ohm ODT Submodel (800/1066Mbps)
DQ_40_ODT30_1066   40 Ohm Data I/O with 30 Ohm ODT Submodel (800/1066Mbps)
DQ_40_ODT40_1066   40 Ohm Data I/O with 40 Ohm ODT Submodel (800/1066Mbps)
DQ_40_ODT60_1066   40 Ohm Data I/O with 60 Ohm ODT Submodel (800/1066Mbps)
DQ_40_ODT120_1066  40 Ohm Data I/O with 120 Ohm ODT Submodel (800/1066Mbps)
DQ_34_1333   34 Ohm Data I/O with no ODT (1333Mbps)
DQ_34_ODT20_1333   34 Ohm Data I/O with 20 Ohm ODT Submodel (1333Mbps)
DQ_34_ODT30_1333   34 Ohm Data I/O with 30 Ohm ODT Submodel (1333Mbps)
DQ_34_ODT40_1333   34 Ohm Data I/O with 40 Ohm ODT Submodel (1333Mbps)
DQ_34_ODT60_1333   34 Ohm Data I/O with 60 Ohm ODT Submodel (1333Mbps)
DQ_34_ODT120_1333  34 Ohm Data I/O with 120 Ohm ODT Submodel (1333Mbps)
DQ_40_1333   40 Ohm Data I/O with no ODT (1333Mbps)
DQ_40_ODT20_1333   40 Ohm Data I/O with 20 Ohm ODT Submodel (1333Mbps)
DQ_40_ODT30_1333   40 Ohm Data I/O with 30 Ohm ODT Submodel (1333Mbps)
DQ_40_ODT40_1333   40 Ohm Data I/O with 40 Ohm ODT Submodel (1333Mbps)
DQ_40_ODT60_1333   40 Ohm Data I/O with 60 Ohm ODT Submodel (1333Mbps)
DQ_40_ODT120_1333  40 Ohm Data I/O with 120 Ohm ODT Submodel (1333Mbps)
DQ_34_1600   34 Ohm Data I/O with no ODT (1600Mbps)
DQ_34_ODT20_1600   34 Ohm Data I/O with 20 Ohm ODT Submodel (1600Mbps)
DQ_34_ODT30_1600   34 Ohm Data I/O with 30 Ohm ODT Submodel (1600Mbps)
DQ_34_ODT40_1600   34 Ohm Data I/O with 40 Ohm ODT Submodel (1600Mbps)
DQ_34_ODT60_1600   34 Ohm Data I/O with 60 Ohm ODT Submodel (1600Mbps)
DQ_34_ODT120_1600  34 Ohm Data I/O with 120 Ohm ODT Submodel (1600Mbps)
DQ_40_1600   40 Ohm Data I/O with no ODT (1600Mbps)
DQ_40_ODT20_1600   40 Ohm Data I/O with 20 Ohm ODT Submodel (1600Mbps)
DQ_40_ODT30_1600   40 Ohm Data I/O with 30 Ohm ODT Submodel (1600Mbps)
DQ_40_ODT40_1600   40 Ohm Data I/O with 40 Ohm ODT Submodel (1600Mbps)
DQ_40_ODT60_1600   40 Ohm Data I/O with 60 Ohm ODT Submodel (1600Mbps)
DQ_40_ODT120_1600  40 Ohm Data I/O with 120 Ohm ODT Submodel (1600Mbps)
DQ_34_2133   34 Ohm Data I/O with no ODT (1866/2133 Mbps)
DQ_34_ODT20_2133   34 Ohm Data I/O with 20 Ohm ODT Submodel (1866/2133 Mbps)
DQ_34_ODT30_2133   34 Ohm Data I/O with 30 Ohm ODT Submodel (1866/2133 Mbps)
DQ_34_ODT40_2133   34 Ohm Data I/O with 40 Ohm ODT Submodel (1866/2133 Mbps)
DQ_34_ODT60_2133   34 Ohm Data I/O with 60 Ohm ODT Submodel (1866/2133 Mbps)
DQ_34_ODT120_2133  34 Ohm Data I/O with 120 Ohm ODT Submodel (1866/2133 Mbps)
DQ_40_2133   40 Ohm Data I/O with no ODT (1866/2133 Mbps)
DQ_40_ODT20_2133   40 Ohm Data I/O with 20 Ohm ODT Submodel (1866/2133 Mbps)
DQ_40_ODT30_2133   40 Ohm Data I/O with 30 Ohm ODT Submodel (1866/2133 Mbps)
DQ_40_ODT40_2133   40 Ohm Data I/O with 40 Ohm ODT Submodel (1866/2133 Mbps)
DQ_40_ODT60_2133   40 Ohm Data I/O with 60 Ohm ODT Submodel (1866/2133 Mbps)
DQ_40_ODT120_2133  40 Ohm Data I/O with 120 Ohm ODT Submodel (1866/2133 Mbps)
[Model Selector] DQS
DQS_34_1066   34 Ohm Strobe I/O with no ODT (800/1066Mbps)
DQS_34_ODT20_1066  34 Ohm Strobe I/O with 20 Ohm ODT Submodel (800/1066Mbps)
DQS_34_ODT30_1066  34 Ohm Strobe I/O with 30 Ohm ODT Submodel (800/1066Mbps)
DQS_34_ODT40_1066  34 Ohm Strobe I/O with 40 Ohm ODT Submodel (800/1066Mbps)
DQS_34_ODT60_1066  34 Ohm Strobe I/O with 60 Ohm ODT Submodel (800/1066Mbps)
DQS_34_ODT120_1066 34 Ohm Strobe I/O with 120 Ohm ODT Submodel (800/1066Mbps)
DQS_40_1066   40 Ohm Strobe I/O with no ODT (800/1066Mbps)
DQS_40_ODT20_1066  40 Ohm Strobe I/O with 20 Ohm ODT Submodel (800/1066Mbps)
DQS_40_ODT30_1066  40 Ohm Strobe I/O with 30 Ohm ODT Submodel (800/1066Mbps)
DQS_40_ODT40_1066  40 Ohm Strobe I/O with 40 Ohm ODT Submodel (800/1066Mbps)
DQS_40_ODT60_1066  40 Ohm Strobe I/O with 60 Ohm ODT Submodel (800/1066Mbps)
DQS_40_ODT120_1066 40 Ohm Strobe I/O with 120 Ohm ODT Submodel (800/1066Mbps)
DQS_34_1333   34 Ohm Strobe I/O with no ODT (1333Mbps)
DQS_34_ODT20_1333  34 Ohm Strobe I/O with 20 Ohm ODT Submodel (1333Mbps)
DQS_34_ODT30_1333  34 Ohm Strobe I/O with 30 Ohm ODT Submodel (1333Mbps)
DQS_34_ODT40_1333  34 Ohm Strobe I/O with 40 Ohm ODT Submodel (1333Mbps)
DQS_34_ODT60_1333  34 Ohm Strobe I/O with 60 Ohm ODT Submodel (1333Mbps)
DQS_34_ODT120_1333 34 Ohm Strobe I/O with 120 Ohm ODT Submodel (1333Mbps)
DQS_40_1333   40 Ohm Strobe I/O with no ODT (1333Mbps)
DQS_40_ODT20_1333  40 Ohm Strobe I/O with 20 Ohm ODT Submodel (1333Mbps)
DQS_40_ODT30_1333  40 Ohm Strobe I/O with 30 Ohm ODT Submodel (1333Mbps)
DQS_40_ODT40_1333  40 Ohm Strobe I/O with 40 Ohm ODT Submodel (1333Mbps)
DQS_40_ODT60_1333  40 Ohm Strobe I/O with 60 Ohm ODT Submodel (1333Mbps)
DQS_40_ODT120_1333 40 Ohm Strobe I/O with 120 Ohm ODT Submodel (1333Mbps)
DQS_34_1600   34 Ohm Strobe I/O with no ODT (1600Mbps)
DQS_34_ODT20_1600  34 Ohm Strobe I/O with 20 Ohm ODT Submodel (1600Mbps)
DQS_34_ODT30_1600  34 Ohm Strobe I/O with 30 Ohm ODT Submodel (1600Mbps)
DQS_34_ODT40_1600  34 Ohm Strobe I/O with 40 Ohm ODT Submodel (1600Mbps)
DQS_34_ODT60_1600  34 Ohm Strobe I/O with 60 Ohm ODT Submodel (1600Mbps)
DQS_34_ODT120_1600 34 Ohm Strobe I/O with 120 Ohm ODT Submodel (1600Mbps)
DQS_40_1600   40 Ohm Strobe I/O with no ODT (1600Mbps)
DQS_40_ODT20_1600  40 Ohm Strobe I/O with 20 Ohm ODT Submodel (1600Mbps)
DQS_40_ODT30_1600  40 Ohm Strobe I/O with 30 Ohm ODT Submodel (1600Mbps)
DQS_40_ODT40_1600  40 Ohm Strobe I/O with 40 Ohm ODT Submodel (1600Mbps)
DQS_40_ODT60_1600  40 Ohm Strobe I/O with 60 Ohm ODT Submodel (1600Mbps)
DQS_40_ODT120_1600 40 Ohm Strobe I/O with 120 Ohm ODT Submodel (1600Mbps)
DQS_34_2133   34 Ohm Strobe I/O with no ODT (1866/2133 Mbps)
DQS_34_ODT20_2133  34 Ohm Strobe I/O with 20 Ohm ODT Submodel (1866/2133 Mbps)
DQS_34_ODT30_2133  34 Ohm Strobe I/O with 30 Ohm ODT Submodel (1866/2133 Mbps)
DQS_34_ODT40_2133  34 Ohm Strobe I/O with 40 Ohm ODT Submodel (1866/2133 Mbps)
DQS_34_ODT60_2133  34 Ohm Strobe I/O with 60 Ohm ODT Submodel (1866/2133 Mbps)
DQS_34_ODT120_2133 34 Ohm Strobe I/O with 120 Ohm ODT Submodel (1866/2133 Mbps)
DQS_40_2133   40 Ohm Strobe I/O with no ODT (1866/2133 Mbps)
DQS_40_ODT20_2133  40 Ohm Strobe I/O with 20 Ohm ODT Submodel (1866/2133 Mbps)
DQS_40_ODT30_2133  40 Ohm Strobe I/O with 30 Ohm ODT Submodel (1866/2133 Mbps)
DQS_40_ODT40_2133  40 Ohm Strobe I/O with 40 Ohm ODT Submodel (1866/2133 Mbps)
DQS_40_ODT60_2133  40 Ohm Strobe I/O with 60 Ohm ODT Submodel (1866/2133 Mbps)
DQS_40_ODT120_2133 40 Ohm Strobe I/O with 120 Ohm ODT Submodel (1866/2133 Mbps)
[Model Selector] DM
DM_INPUT_1066   DM Input Model with no ODT (800/1066Mbps)
DM_ODT20_1066   DM Input Model with 20 ohm ODT (800/1066Mbps)
DM_ODT30_1066   DM Input Model with 30 ohm ODT (800/1066Mbps)
DM_ODT40_1066   DM Input Model with 40 ohm ODT (800/1066Mbps)
DM_ODT60_1066   DM Input Model with 60 ohm ODT (800/1066Mbps)
DM_ODT120_1066   DM Input Model with 120 ohm ODT (800/1066Mbps)
DM_INPUT_1600   DM Input Model with no ODT (1600Mbps)
DM_ODT20_1600   DM Input Model with 20 ohm ODT (1600Mbps)
DM_ODT30_1600   DM Input Model with 30 ohm ODT (1600Mbps)
DM_ODT40_1600   DM Input Model with 40 ohm ODT (1600Mbps)
DM_ODT60_1600   DM Input Model with 60 ohm ODT (1600Mbps)
DM_ODT120_1600   DM Input Model with 120 ohm ODT (1600Mbps)
DM_INPUT_1333   DM Input Model with no ODT (1333Mbps)
DM_ODT20_1333   DM Input Model with 20 ohm ODT (1333Mbps)
DM_ODT30_1333   DM Input Model with 30 ohm ODT (1333Mbps)
DM_ODT40_1333   DM Input Model with 40 ohm ODT (1333Mbps)
DM_ODT60_1333   DM Input Model with 60 ohm ODT (1333Mbps)
DM_ODT120_1333   DM Input Model with 120 ohm ODT (1333Mbps)
DM_INPUT_2133   DM Input Model with no ODT (1866/2133 Mbps)
DM_ODT20_2133   DM Input Model with 20 ohm ODT (1866/2133 Mbps)
DM_ODT30_2133   DM Input Model with 30 ohm ODT (1866/2133 Mbps)
DM_ODT40_2133   DM Input Model with 40 ohm ODT (1866/2133 Mbps)
DM_ODT60_2133   DM Input Model with 60 ohm ODT (1866/2133 Mbps)
DM_ODT120_2133   DM Input Model with 120 ohm ODT (1866/2133 Mbps)
[Model Selector] DM_TDQS
DM_INPUT_1066   DM Input Model with no ODT (800/1066Mbps)
DM_ODT20_1066   DM Input Model with 20 ohm ODT (800/1066Mbps)
DM_ODT30_1066   DM Input Model with 30 ohm ODT (800/1066Mbps)
DM_ODT40_1066   DM Input Model with 40 ohm ODT (800/1066Mbps)
DM_ODT60_1066   DM Input Model with 60 ohm ODT (800/1066Mbps)
DM_ODT120_1066   DM Input Model with 120 ohm ODT (800/1066Mbps)
DM_INPUT_1333   DM Input Model with no ODT (1333Mbps)
DM_ODT20_1333   DM Input Model with 20 ohm ODT (1333Mbps)
DM_ODT30_1333   DM Input Model with 30 ohm ODT (1333Mbps)
DM_ODT40_1333   DM Input Model with 40 ohm ODT (1333Mbps)
DM_ODT60_1333   DM Input Model with 60 ohm ODT (1333Mbps)
DM_ODT120_1333   DM Input Model with 120 ohm ODT (1333Mbps)
DM_INPUT_1600   DM Input Model with no ODT (1600Mbps)
DM_ODT20_1600   DM Input Model with 20 ohm ODT (1600Mbps)
DM_ODT30_1600   DM Input Model with 30 ohm ODT (1600Mbps)
DM_ODT40_1600   DM Input Model with 40 ohm ODT (1600Mbps)
DM_ODT60_1600   DM Input Model with 60 ohm ODT (1600Mbps)
DM_ODT120_1600   DM Input Model with 120 ohm ODT (1600Mbps)
DM_INPUT_2133   DM Input Model with no ODT (1866/2133 Mbps)
DM_ODT20_2133   DM Input Model with 20 ohm ODT (1866/2133 Mbps)
DM_ODT30_2133   DM Input Model with 30 ohm ODT (1866/2133 Mbps)
DM_ODT40_2133   DM Input Model with 40 ohm ODT (1866/2133 Mbps)
DM_ODT60_2133   DM Input Model with 60 ohm ODT (1866/2133 Mbps)
DM_ODT120_2133   DM Input Model with 120 ohm ODT (1866/2133 Mbps)
TDQS_ODT20_1066   TDQS Termination Model with 20 ohm ODT (800/1066Mbps)
TDQS_ODT30_1066   TDQS Termination Model with 30 ohm ODT (800/1066Mbps)
TDQS_ODT40_1066   TDQS Termination Model with 40 ohm ODT (800/1066Mbps)
TDQS_ODT60_1066   TDQS Termination Model with 60 ohm ODT (800/1066Mbps)
TDQS_ODT120_1066   TDQS Termination Model with 120 ohm ODT (800/1066Mbps)
TDQS_ODT20_1333   TDQS Termination Model with 20 ohm ODT (1333Mbps)
TDQS_ODT30_1333   TDQS Termination Model with 30 ohm ODT (1333Mbps)
TDQS_ODT40_1333   TDQS Termination Model with 40 ohm ODT (1333Mbps)
TDQS_ODT60_1333   TDQS Termination Model with 60 ohm ODT (1333Mbps)
TDQS_ODT120_1333   TDQS Termination Model with 120 ohm ODT (1333Mbps)
TDQS_ODT20_1600   TDQS Termination Model with 20 ohm ODT (1600Mbps)
TDQS_ODT30_1600   TDQS Termination Model with 30 ohm ODT (1600Mbps)
TDQS_ODT40_1600   TDQS Termination Model with 40 ohm ODT (1600Mbps)
TDQS_ODT60_1600   TDQS Termination Model with 60 ohm ODT (1600Mbps)
TDQS_ODT120_1600   TDQS Termination Model with 120 ohm ODT (1600Mbps)
TDQS_ODT20_2133   TDQS Termination Model with 20 ohm ODT (1866/2133 Mbps)
TDQS_ODT30_2133   TDQS Termination Model with 30 ohm ODT (1866/2133 Mbps)
TDQS_ODT40_2133   TDQS Termination Model with 40 ohm ODT (1866/2133 Mbps)
TDQS_ODT60_2133   TDQS Termination Model with 60 ohm ODT (1866/2133 Mbps)
TDQS_ODT120_2133   TDQS Termination Model with 120 ohm ODT (1866/2133 Mbps)
[Model Selector] NF_TDQS#
TDQS_ODT20_1066   TDQS Termination Model with 20 ohm ODT (800/1066Mbps)
TDQS_ODT30_1066   TDQS Termination Model with 30 ohm ODT (800/1066Mbps)
TDQS_ODT40_1066   TDQS Termination Model with 40 ohm ODT (800/1066Mbps)
TDQS_ODT60_1066   TDQS Termination Model with 60 ohm ODT (800/1066Mbps)
TDQS_ODT120_1066   TDQS Termination Model with 120 ohm ODT (800/1066Mbps)
TDQS_ODT20_1333   TDQS Termination Model with 20 ohm ODT (1333Mbps)
TDQS_ODT30_1333   TDQS Termination Model with 30 ohm ODT (1333Mbps)
TDQS_ODT40_1333   TDQS Termination Model with 40 ohm ODT (1333Mbps)
TDQS_ODT60_1333   TDQS Termination Model with 60 ohm ODT (1333Mbps)
TDQS_ODT120_1333   TDQS Termination Model with 120 ohm ODT (1333Mbps)
TDQS_ODT20_1600   TDQS Termination Model with 20 ohm ODT (1600Mbps)
TDQS_ODT30_1600   TDQS Termination Model with 30 ohm ODT (1600Mbps)
TDQS_ODT40_1600   TDQS Termination Model with 40 ohm ODT (1600Mbps)
TDQS_ODT60_1600   TDQS Termination Model with 60 ohm ODT (1600Mbps)
TDQS_ODT120_1600   TDQS Termination Model with 120 ohm ODT (1600Mbps)
TDQS_ODT20_2133   TDQS Termination Model with 20 ohm ODT (1866/2133 Mbps)
TDQS_ODT30_2133   TDQS Termination Model with 30 ohm ODT (1866/2133 Mbps)
TDQS_ODT40_2133   TDQS Termination Model with 40 ohm ODT (1866/2133 Mbps)
TDQS_ODT60_2133   TDQS Termination Model with 60 ohm ODT (1866/2133 Mbps)
TDQS_ODT120_2133   TDQS Termination Model with 120 ohm ODT (1866/2133 Mbps)
NF_INPUT   Non-functioning input (NF)
[Model Selector] TDQS
TDQS_ODT20_1066   TDQS Termination Model with 20 ohm ODT (800/1066Mbps)
TDQS_ODT30_1066   TDQS Termination Model with 30 ohm ODT (800/1066Mbps)
TDQS_ODT40_1066   TDQS Termination Model with 40 ohm ODT (800/1066Mbps)
TDQS_ODT60_1066   TDQS Termination Model with 60 ohm ODT (800/1066Mbps)
TDQS_ODT120_1066   TDQS Termination Model with 120 ohm ODT (800/1066Mbps)
TDQS_ODT20_1333   TDQS Termination Model with 20 ohm ODT (1333Mbps)
TDQS_ODT30_1333   TDQS Termination Model with 30 ohm ODT (1333Mbps)
TDQS_ODT40_1333   TDQS Termination Model with 40 ohm ODT (1333Mbps)
TDQS_ODT60_1333   TDQS Termination Model with 60 ohm ODT (1333Mbps)
TDQS_ODT120_1333   TDQS Termination Model with 120 ohm ODT (1333Mbps)
TDQS_ODT20_1600   TDQS Termination Model with 20 ohm ODT (1600Mbps)
TDQS_ODT30_1600   TDQS Termination Model with 30 ohm ODT (1600Mbps)
TDQS_ODT40_1600   TDQS Termination Model with 40 ohm ODT (1600Mbps)
TDQS_ODT60_1600   TDQS Termination Model with 60 ohm ODT (1600Mbps)
TDQS_ODT120_1600   TDQS Termination Model with 120 ohm ODT (1600Mbps)
TDQS_ODT20_2133   TDQS Termination Model with 20 ohm ODT (1866/2133 Mbps)
TDQS_ODT30_2133   TDQS Termination Model with 30 ohm ODT (1866/2133 Mbps)
TDQS_ODT40_2133   TDQS Termination Model with 40 ohm ODT (1866/2133 Mbps)
TDQS_ODT60_2133   TDQS Termination Model with 60 ohm ODT (1866/2133 Mbps)
TDQS_ODT120_2133   TDQS Termination Model with 120 ohm ODT (1866/2133 Mbps)
[Model Selector] INPUT
INPUT_1066   Address/Command/Control Input model (800/1066Mbps)
INPUT_1333   Address/Command/Control Input model (1333Mbps)
INPUT_1600   Address/Command/Control Input model (1600Mbps)
INPUT_2133   Address/Command/Control Input model (1866/2133 Mbps)
[Model Selector] CLKIN
CLKIN_1066   Clock Input model (800/1066Mbps)
CLKIN_1333   Clock Input model (1333Mbps)
CLKIN_1600   Clock Input model (1600Mbps)
CLKIN_2133   Clock Input model (1866/2133 Mbps)
[Model Selector] ODT_INPUT
ODT_INPUT_1066   ODT Input model (800/1066Mbps)
ODT_INPUT_1333   ODT Input model (1333Mbps)
ODT_INPUT_1600   ODT Input model (1600Mbps)
ODT_INPUT_2133   ODT Input model (1866/2133 Mbps)
| Sparse Matrix Package Model for v69a_78ball_pkg (x4/x8)
[Define Package Model]  V69A_X4_X8_FULL_PKG
[Manufacturer]   Micron Technology, Inc.
[OEM]   Micron Technology, Inc.
[Description]   78B 9X11.5mm BGA
[Number of Pins]   69
[Pin Numbers]
A1
A2
A7
A8
A9
B2
B3
B7
B8
B9
C1
C2
C3
C7
C8
C9
D1
D2
D3
D7
D8
E1
E2
E3
E7
E8
E9
F1
F2
F3
F7
F8
F9
G1
G2
G3
G7
G8
G9
H1
H2
H3
H7
H8
H9
J1
J2
J3
J8
J9
K1
K2
K3
K7
K8
L2
L3
L7
L8
M1
M2
M3
M7
M8
M9
N2
N3
N7
N8
[Model Data]
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[End Model Data]
[End Package Model]
| Sparse Matrix Package Model for v69a_96ball_pkg (x4/x8)
[Define Package Model]  V69A_X16_FULL_PKG
[Manufacturer]   Micron Technology, Inc.
[OEM]   Micron Technology, Inc.
[Description]  96B 9x14.0mm BGA
[Number of Pins]   86
[Pin Numbers]
A1
A2
A3
A7
A8
B1
B2
B3
B7
B8
B9
C1
C2
C3
C7
C8
C9
D1
D2
D3
D7
D8
D9
E1
E2
E3
E7
E8
F1
F2
F3
F7
F8
G2
G3
G7
G8
G9
H1
H2
H3
H7
H8
H9
J1
J2
J3
J7
J8
J9
K1
K2
K3
K7
K8
K9
L1
L2
L3
L7
L8
L9
M1
M2
M3
M8
N1
N2
N3
N7
N8
N9
P2
P3
P7
P8
R1
R2
R3
R7
R8
T1
T2
T3
T7
T8
[Model Data]
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[End Model Data]
[End Package Model]
| Models and submodels in the file (173): DQ_34_1066 (I/O), DQ_34_ODT20_1066 (I/O), DQ_34_ODT30_1066 (I/O), DQ_34_ODT40_1066 (I/O), DQ_34_ODT60_1066 (I/O), DQ_34_ODT120_1066 (I/O), DQ_40_1066 (I/O), DQ_40_ODT20_1066 (I/O), DQ_40_ODT30_1066 (I/O), DQ_40_ODT40_1066 (I/O), DQ_40_ODT60_1066 (I/O), DQ_40_ODT120_1066 (I/O), DQ_34_1333 (I/O), DQ_34_ODT20_1333 (I/O), DQ_34_ODT30_1333 (I/O), DQ_34_ODT40_1333 (I/O), DQ_34_ODT60_1333 (I/O), DQ_34_ODT120_1333 (I/O), DQ_40_1333 (I/O), DQ_40_ODT20_1333 (I/O), DQ_40_ODT30_1333 (I/O), DQ_40_ODT40_1333 (I/O), DQ_40_ODT60_1333 (I/O), DQ_40_ODT120_1333 (I/O), DQ_34_1600 (I/O), DQ_34_ODT20_1600 (I/O), DQ_34_ODT30_1600 (I/O), DQ_34_ODT40_1600 (I/O), DQ_34_ODT60_1600 (I/O), DQ_34_ODT120_1600 (I/O), DQ_40_1600 (I/O), DQ_40_ODT20_1600 (I/O), DQ_40_ODT30_1600 (I/O), DQ_40_ODT40_1600 (I/O), DQ_40_ODT60_1600 (I/O), DQ_40_ODT120_1600 (I/O), DQ_34_2133 (I/O), DQ_34_ODT20_2133 (I/O), DQ_34_ODT30_2133 (I/O), DQ_34_ODT40_2133 (I/O), DQ_34_ODT60_2133 (I/O), DQ_34_ODT120_2133 (I/O), DQ_40_2133 (I/O), DQ_40_ODT20_2133 (I/O), DQ_40_ODT30_2133 (I/O), DQ_40_ODT40_2133 (I/O), DQ_40_ODT60_2133 (I/O), DQ_40_ODT120_2133 (I/O), DQS_34_1066 (I/O), DQS_34_ODT20_1066 (I/O), DQS_34_ODT30_1066 (I/O), DQS_34_ODT40_1066 (I/O), DQS_34_ODT60_1066 (I/O), DQS_34_ODT120_1066 (I/O), DQS_40_1066 (I/O), DQS_40_ODT20_1066 (I/O), DQS_40_ODT30_1066 (I/O), DQS_40_ODT40_1066 (I/O), DQS_40_ODT60_1066 (I/O), DQS_40_ODT120_1066 (I/O), DQS_34_1333 (I/O), DQS_34_ODT20_1333 (I/O), DQS_34_ODT30_1333 (I/O), DQS_34_ODT40_1333 (I/O), DQS_34_ODT60_1333 (I/O), DQS_34_ODT120_1333 (I/O), DQS_40_1333 (I/O), DQS_40_ODT20_1333 (I/O), DQS_40_ODT30_1333 (I/O), DQS_40_ODT40_1333 (I/O), DQS_40_ODT60_1333 (I/O), DQS_40_ODT120_1333 (I/O), DQS_34_1600 (I/O), DQS_34_ODT20_1600 (I/O), DQS_34_ODT30_1600 (I/O), DQS_34_ODT40_1600 (I/O), DQS_34_ODT60_1600 (I/O), DQS_34_ODT120_1600 (I/O), DQS_40_1600 (I/O), DQS_40_ODT20_1600 (I/O)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
